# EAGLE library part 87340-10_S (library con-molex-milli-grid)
RECEPTACAL
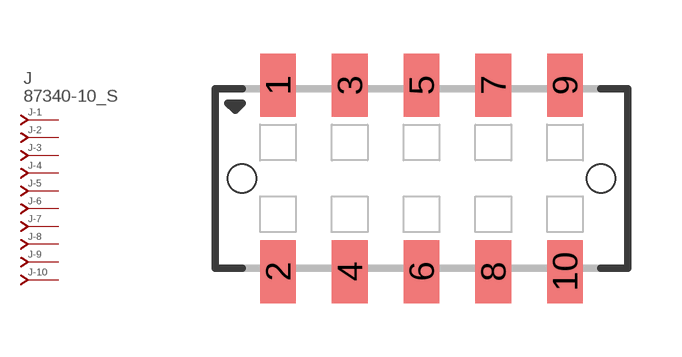
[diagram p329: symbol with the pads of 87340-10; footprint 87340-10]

Designator prefix J; gates -1=J-NV -2=J-N -3=J-N -4=J-N -5=J-N -6=J-N -7=J-N -8=J-N -9=J-N -10=J-N

## 87340-10_S  [87340-10]
1  -1:J  pas
2  -2:J  pas
3  -3:J  pas
4  -4:J  pas
5  -5:J  pas
6  -6:J  pas
7  -7:J  pas
8  -8:J  pas
9  -9:J  pas
10  -10:J  pas

## Footprint 87340-10 (pad centres in mm)
RECEPTACAL SMD Dual Row, Vertical, Low Profile
smd 1 x 1.75: 1 -4,2.6; 2 -4,-2.6; 3 -2,2.6; 4 -2,-2.6; 5 0,2.6; 6 0,-2.6; 7 2,2.6; 8 2,-2.6; 9 4,2.6; 10 4,-2.6
hole 0.8 at -5,0
hole 0.8 at 5,0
